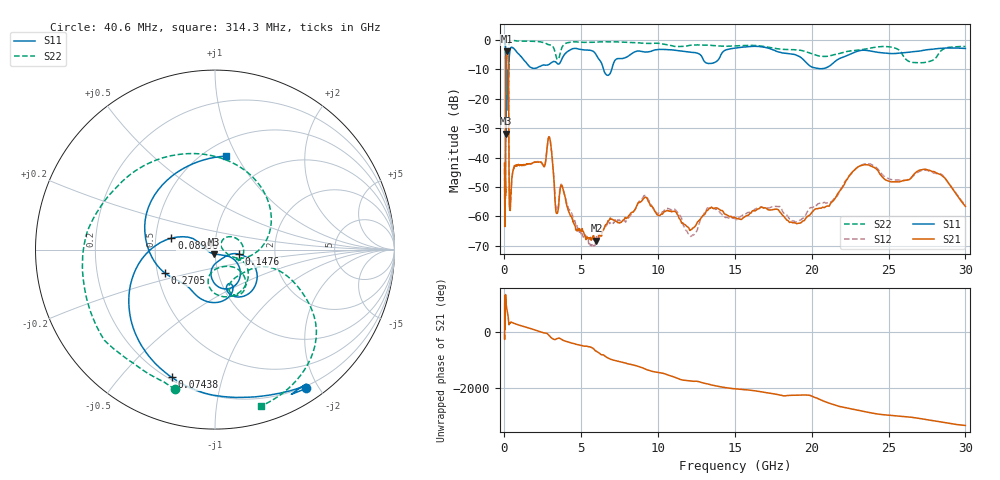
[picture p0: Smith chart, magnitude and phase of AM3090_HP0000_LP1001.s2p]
! Date/Time: Thu, Feb 28, 2019 1:53 PM
! Network Analyzer: Agilent Technologies E8364B Rev: A.07.50.67
! Sweep from 0.010 to 30.000 GHz, 1601 Points, Sweep Type: LOG
! Power Supply: 5.022 V, 0.002 A
# Hz S DB R 50
!freq MagS11 AngS11 MagS21 AngS21 MagS12 AngS12 MagS22 AngS22
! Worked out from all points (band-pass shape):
!   1601 points, 10 MHz to 30 GHz, reference 50 ohm
!   highest |S21| = -3.79 dB at 147.6 MHz (marker M1); lowest = -68.2 dB at 5.989 GHz (marker M2)
!   |S21| within 3 dB of the highest: 99.26 MHz to 248.6 MHz (149.3 MHz wide, 85.9 % of centre)
!   lowest |S11| = -31.8 dB at 97.94 MHz (marker M3), VSWR 1.05, Z = 49.2 - j2.42 ohm
!   |S11| at or under -10 dB: 88.91 MHz to 271.7 MHz (182.8 MHz wide, 101 % of centre); 6.454 GHz to 6.98 GHz (525.8 MHz wide, 7.83 % of centre)
!   |S22| runs from -28.3 to -0.1 dB; largest |S21 - S12| = 0.012
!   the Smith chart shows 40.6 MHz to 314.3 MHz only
!   S11 on the Smith chart (normalised r, x): 40.6 MHz: 0.17, -1.84; 74.38 MHz: 0.21, -0.70; 89.96 MHz: 0.61, +0.08; 147.6 MHz: 1.31, -0.07; 270.5 MHz: 0.55, -0.16; 314.3 MHz: 0.63, +0.90
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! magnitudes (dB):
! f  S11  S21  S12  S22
! 10 MHz  -0.2  -41.9  -45.5  -0.6
! 38.04 MHz  -0.5  -57.8  -59.3  -1.6
! 40.6 MHz  -0.7  -60.5  -59.8  -1.8
! 74.38 MHz  -2.5  -44.6  -46.8  -4.5
! 89.96 MHz  -12.0  -14.4  -14.3  -11.7
! 97.94 MHz  -31.8  -7.2  -7.2  -27.1
! 114.4 MHz  -12.9  -4.8  -4.8  -17.7
! 144.7 MHz  -20.0  -3.8  -3.8  -17.2
! 147.6 MHz  -17.2  -3.8  -3.8  -16.5
! 237.5 MHz  -10.7  -5.8  -5.8  -10.9
! 270.5 MHz  -10.2  -14.0  -14.0  -9.4
! 314.3 MHz  -5.6  -53.8  -54.6  -0.8
! 550.5 MHz  -2.7  -44.7  -44.6  -0.2
! 2.084 GHz  -9.5  -41.5  -41.4  -0.5
! 2.928 GHz  -8.2  -33.1  -33.1  -1.6
! 3.402 GHz  -7.8  -58.9  -58.0  -6.3
! 3.76 GHz  -6.2  -49.8  -49.5  -2.3
! 5.989 GHz  -5.2  -68.2  -66.8  -0.7
! 7.926 GHz  -5.9  -60.7  -61.4  -0.7
! 19.12 GHz  -5.4  -62.3  -61.7  -3.4
! 23.48 GHz  -3.5  -42.4  -42.1  -3.1
! 30 GHz  -2.8  -56.6  -56.1  -2.2
